FUNCTION_BLOCK FB_GeneratorEX EXTENDS FB_Generator
VAR_INPUT
END_VAR
VAR_OUTPUT
END_VAR
VAR
END_VAR

{warning 'add method implementation'}
METHOD M_Flash : BOOL
fbTon1(IN:=NOT fbTon1.Q , 
		PT:=tCycletime , 
		Q=> , ET=> );

// 33% ON 66% OFF
M_Flash := fbTon1.ET < fbTon1.PT / 3 ;
END_METHOD

PROPERTY P_Vendor : STRING
GET
P_Vendor := CONCAT(STR1:='Company Y based on ' , 
       			 STR2:=SUPER^.P_Vendor );
END_GET
END_PROPERTY

END_FUNCTION_BLOCK
